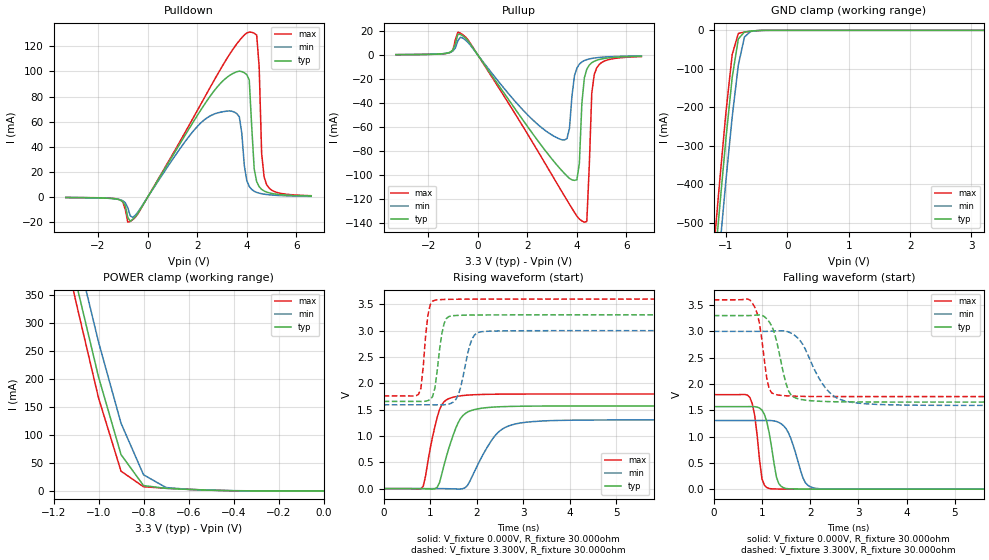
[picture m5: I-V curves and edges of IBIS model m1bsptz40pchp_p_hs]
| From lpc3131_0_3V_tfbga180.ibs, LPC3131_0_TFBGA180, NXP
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| |   Rev 0.20 IBIS Model Design Automation Generation   |
| |   N O N - S I L I C O N   C O R R E L A T E D   |
| |   This IBIS [Model] is pre-Beta tactical support   |
| |  Note: this IBIS [Model] contains clamp curves generated   |
| |   through simulation which should not be relied upon   |
| Date/Time   : 2010 Jan 25 (Mon) 11:58:19
| Pccmos090 jliolib_p50 2.0
|   0.9 um 3.3V pad library
|   seven level metal
|   dual oxide
|   dual threshold voltage
|   nominal line mixed supply
|   parasitic extracted netlists
| Process block a10
| mem1bsptz40pchp
|   Bidirectional Pad 3.3
|   3state Output
|   Plain Input
|   CMOS
|   Programmable between
|   - (p1=0, p2=1) plain input
|   - (p1=0, p2=0) with Pull Up
|   - (p1=1, p2=1) with Pull Down
|   - (p1=1, p2=0) with Repeater
| Plain input Mode high speed (esh=0, p1=0, p2=1)
[Model]   m1bsptz40pchp_p_hs | of mem1bsptz40pchp
Model_type   I/O
Polarity   Non-Inverting
Enable   Active-Low
|  Reciever Thresholds
Vinl   = 0.99V
Vinh   = 2.31V
| AC Test Load Conditions
Vref   = 0
Cref   = 0
Rref   = 1000000000
Vmeas   = 1.65
| [Process Range]   typical   min   max
| C_comp edge width   400.000ps   400.000ps   400.000ps
| C_comp Tstrobe   40.000fs   40.000fs   40.000fs
C_comp   200.000pF   200.000pF   200.000pF
[Temperature Range]   25   125   -40
[Voltage Range]   3.30V   3.00V   3.60V
[GND Clamp Reference]   0.00V   0.00V   0.00V
[Pulldown Reference]   0.00V   0.00V   0.00V
[POWER Clamp Reference]   3.30V   3.00V   3.60V
[Pullup Reference]   3.30V   3.00V   3.60V
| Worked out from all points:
|   slope of the pulldown table from 0 to 0.495 V, typ, clamps not added: 30.7 ohm
|   slope of the pullup table from 0 to 0.495 V, typ, clamps not added: 33.2 ohm
|   GND clamp passes 1 mA (typ) near -0.52 V on its own axis
|   POWER clamp passes 1 mA (typ) near -0.48 V on its own axis
|   rising waveform, V_fixture 0.000V, R_fixture 30.000ohm: 20-80 % time 343ps typ, 516ps min, 257ps max; typ from 0 V to 1.57 V
|   falling waveform, V_fixture 0.000V, R_fixture 30.000ohm: 20-80 % time 177ps typ, 272ps min, 137ps max; typ from 1.57 V to 0 V
|   rising waveform, V_fixture 3.300V, R_fixture 30.000ohm: 20-80 % time 145ps typ, 213ps min, 115ps max; typ from 1.66 V to 3.3 V
|   falling waveform, V_fixture 3.300V, R_fixture 30.000ohm: 20-80 % time 251ps typ, 500ps min, 169ps max; typ from 3.3 V to 1.66 V
[GND Clamp]
| ref voltage   0.00V   0.00V   0.00V
|   Voltage   I(typ)   I(min)   I(max)
-3.3V     -4.732A    -4.814A    -4.684A
-1.2V     -636mA     -742.5mA   -569.7mA
-1.1V     -453.5mA   -561.8mA   -385.7mA
-1V       -279mA     -387.5mA   -210.8mA
-900mV    -122.8mA   -225.5mA   -63.11mA
-800mV    -22.42mA   -90.48mA   -8.158mA
-700mV    -4.346mA   -17.29mA   -4.479mA
-600mV    -2.103mA   -3.017mA   -2.46mA
-300mV    -3.346uA   -19.56uA   -987.1nA
3.2V      182pA      6.98uA     191.9pA
[Power Clamp]   | Vtable = Vcc - Vpad
| ref voltage   3.30V   3.00V   3.60V
|   Voltage   I(typ)   I(min)   I(max)
-3.3V     4.647A     4.675A     4.636A
-1.2V     553.3mA    610.4mA    520.8mA
-1.1V     373.2mA    433.6mA    337.9mA
-1V       204mA      266.6mA    166.4mA
-900mV    65.06mA    121.2mA    35.38mA
-800mV    9.603mA    28.92mA    7.422mA
-700mV    4.54mA     6.054mA    4.861mA
-600mV    2.669mA    2.794mA    2.852mA
-400mV    308.1uA    509.7uA    227.2uA
0V        393.8pA    9.961nA    269.9pA
[Pulldown]
| ref voltage   0.00V   0.00V   0.00V
|   Voltage   I(typ)   I(min)   I(max)
-3.3V     -236.8uA   -252.6uA   -192.2uA
-1.2V     -1.654mA   -1.557mA   -1.498mA
-600mV    -17.59mA   -16.04mA   -17.81mA
2.9V      89.68mA    67.41mA    100.4mA
3.7V      100.2mA    63.84mA    124.5mA
4.1V      93.21mA    8.525mA    131.3mA
4.3V      22.46mA    4.748mA    130.4mA
4.4V      12.41mA    3.864mA    128.9mA
4.5V      8.379mA    3.247mA    103.7mA
4.6V      6.229mA    2.794mA    34.8mA
4.8V      4.116mA    2.178mA    10.07mA
6.6V      977.1uA    710.9uA    1.218mA
[Pullup]   | Vtable = Vcc - Vpad
| ref voltage   3.30V   3.00V   3.60V
|   Voltage   I(typ)   I(min)   I(max)
-3.3V     206.9uA    209uA      174.2uA
-500mV    14.09mA    12.45mA    15.05mA
3.4V      -96.53mA   -70.69mA   -114.1mA
3.7V      -102.8mA   -61.23mA   -124.3mA
3.9V      -104.5mA   -17.63mA   -131mA
4.1V      -90.2mA    -7.678mA   -136.7mA
4.2V      -40.59mA   -5.874mA   -138.2mA
4.3V      -19.19mA   -4.731mA   -139.3mA
4.4V      -11.92mA   -3.949mA   -138.6mA
4.6V      -6.518mA   -2.953mA   -31.79mA
4.7V      -5.293mA   -2.618mA   -16.38mA
6.6V      -1.121mA   -811.3uA   -1.417mA
[Ramp]
R_load   = 30.000ohm
|   dV/dt(typ)   dV/dt(min)   dV/dt(max)
dV/dt_r   941.610mV/350.000ps   782.836mV/500.000ps   1.078V/250.000ps
dV/dt_f   986.369mV/250.000ps   844.783mV/500.000ps   1.104V/150.000ps
[Rising Waveform]  | cubic spline decimation from 501 points
V_fixture   = 0.000V
R_fixture   = 30.000ohm
|   Time   V(typ)   V(min)   V(max)
0s        4.028nV    182.8nV    2.848nV
850ps     -1.566mV   23.17uV    44.26mV
1.15ns    23.73mV    142.9uV    1.353V
1.35ns    616.1mV    -1.77mV    1.686V
1.6ns     1.251V     -8.255mV   1.755V
1.75ns    1.424V     16.91mV    1.772V
2.25ns    1.541V     821.9mV    1.791V
2.5ns     1.555V     1.099V     1.794V
3.4ns     1.568V     1.284V     1.797V
25ns      1.569V     1.305V     1.797V
[Falling Waveform]  | cubic spline decimation from 501 points
V_fixture   = 0.000V
R_fixture   = 30.000ohm
|   Time   V(typ)   V(min)   V(max)
0s        1.569V     1.305V     1.797V
750ps     1.57V      1.305V     1.741V
850ps     1.568V     1.305V     1.394V
1ns       1.503V     1.305V     196.1mV
1.2ns     792.4mV    1.303V     6.933mV
1.3ns     227.9mV    1.287V     3.831mV
1.4ns     51.85mV    1.242V     2.21mV
1.9ns     1.354mV    122.7mV    244.3uV
2.2ns     465.3uV    7.616mV    88.41uV
25ns      30.82nV    223.1nV    -51.71nV
[Rising Waveform]  | cubic spline decimation from 501 points
V_fixture   = 3.300V
V_fixture_min = 3.000V
V_fixture_max = 3.600V
R_fixture   = 30.000ohm
|   Time   V(typ)   V(min)   V(max)
0s        1.656V     1.592V     1.76V
750ps     1.656V     1.592V     1.792V
800ps     1.655V     1.592V     1.904V
950ps     1.671V     1.592V     3.289V
1.15ns    2.236V     1.591V     3.585V
1.35ns    3.232V     1.597V     3.594V
1.6ns     3.29V      1.774V     3.597V
1.9ns     3.297V     2.843V     3.599V
2.2ns     3.298V     2.987V     3.599V
25ns      3.3V       3V         3.6V
[Falling Waveform]  | cubic spline decimation from 501 points
V_fixture   = 3.300V
V_fixture_min = 3.000V
V_fixture_max = 3.600V
R_fixture   = 30.000ohm
|   Time   V(typ)   V(min)   V(max)
0s        3.3V       3V         3.6V
800ps     3.303V     3V         3.54V
950ps     3.313V     3V         3.14V
1.15ns    3.181V     3.002V     1.904V
1.3ns     2.827V     3.009V     1.796V
1.45ns    2.186V     3.01V      1.778V
1.65ns    1.755V     2.942V     1.768V
2.45ns    1.663V     1.798V     1.76V
3.15ns    1.657V     1.623V     1.76V
25ns      1.656V     1.592V     1.76V
